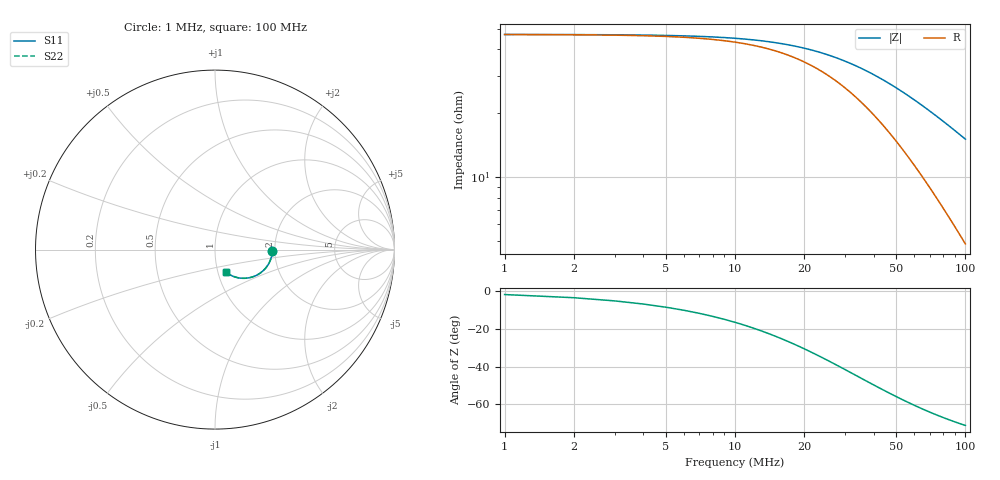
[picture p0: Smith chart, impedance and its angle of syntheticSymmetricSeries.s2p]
# MHz S RI R 50.0000
! SimSmith 18.3b
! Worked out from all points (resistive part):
!   100 points, 1 MHz to 100 MHz, reference 50 ohm
!   read as one part in series: R = 47 ohm at 1 MHz
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1  0.3196 -0.00642  0.6804 0.00642  0.6804 0.00642  0.3196 -0.00642
3  0.3186 -0.0192  0.6814 0.0192  0.6814 0.0192  0.3186 -0.0192
5  0.3165 -0.0318  0.6835 0.0318  0.6835 0.0318  0.3165 -0.0318
9  0.3096 -0.056  0.6904 0.056  0.6904 0.056  0.3096 -0.056
11  0.3048 -0.0674  0.6952 0.0674  0.6952 0.0674  0.3048 -0.0674
14  0.2963 -0.0833  0.7037 0.0833  0.7037 0.0833  0.2963 -0.0833
18  0.2828 -0.1022  0.7172 0.1022  0.7172 0.1022  0.2828 -0.1022
22  0.2675 -0.1182  0.7325 0.1182  0.7325 0.1182  0.2675 -0.1182
26  0.2512 -0.1312  0.7488 0.1312  0.7488 0.1312  0.2512 -0.1312
30  0.2345 -0.1414  0.7655 0.1414  0.7655 0.1414  0.2345 -0.1414
34  0.218 -0.1489  0.782 0.1489  0.782 0.1489  0.218 -0.1489
38  0.202 -0.1542  0.798 0.1542  0.798 0.1542  0.202 -0.1542
42  0.1868 -0.1576  0.8132 0.1576  0.8132 0.1576  0.1868 -0.1576
46  0.1725 -0.1594  0.8275 0.1594  0.8275 0.1594  0.1725 -0.1594
51  0.156 -0.1598  0.844 0.1598  0.844 0.1598  0.156 -0.1598
55  0.144 -0.1591  0.856 0.1591  0.856 0.1591  0.144 -0.1591
59  0.133 -0.1576  0.867 0.1576  0.867 0.1576  0.133 -0.1576
67  0.1137 -0.1531  0.8863 0.1531  0.8863 0.1531  0.1137 -0.1531
75  0.0978 -0.1473  0.9022 0.1473  0.9022 0.1473  0.0978 -0.1473
84  0.0831 -0.1402  0.9169 0.1402  0.9169 0.1402  0.0831 -0.1402
92  0.0724 -0.1338  0.9276 0.1338  0.9276 0.1338  0.0724 -0.1338
100  0.0635 -0.1275  0.9365 0.1275  0.9365 0.1275  0.0635 -0.1275
